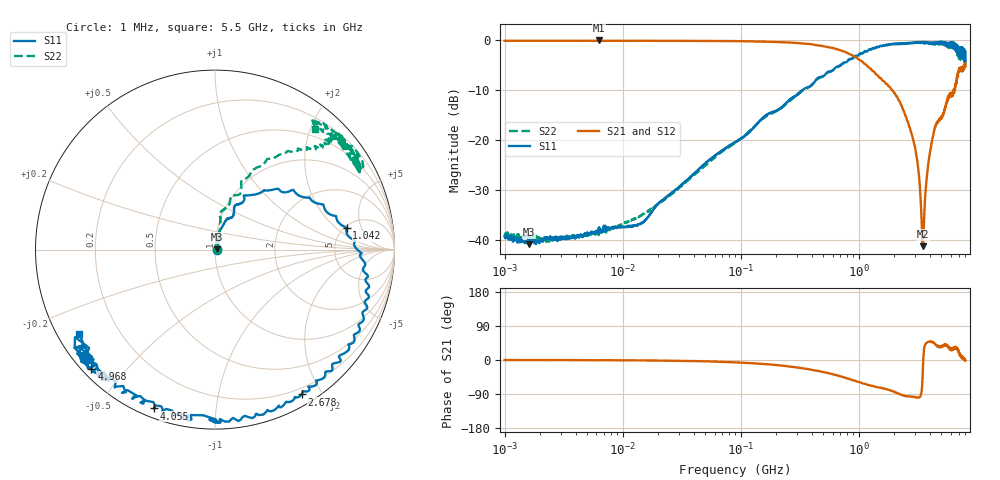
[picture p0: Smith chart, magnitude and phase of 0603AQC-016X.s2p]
!s-Parameter Generated by FASTRON Sdn. Bhd.
!FASTRON P/N : 0603AQC-016X
!Keysight Technologies: E5071C_MY46733604_B.14.02
!Date: Thu Jun 25 13:52:09 2026
!Version  :Rev00  Thu Jun 25 13:52:09 2026
!Data & Calibration Information:
!Freq  S11:SOLT2(ON)  S21:SOLT2(ON)  S12:SOLT2(ON)  S22:SOLT2(ON)
!PortZ  Port1:50+j0  Port2:50+j0
!When reading reference impedance value at option line is always used.
! Remarks : This data is being provided solely for informational purposes.
# Hz S dB R 50
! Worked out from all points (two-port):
!   1601 points, 1 MHz to 8 GHz, reference 50 ohm
!   highest |S21| = -0.03 dB at 6.268 MHz (marker M1); lowest = -41.2 dB at 3.487 GHz (marker M2)
!   |S21| within 3 dB of the highest: start of sweep to 884.1 MHz
!   lowest |S11| = -40.8 dB at 1.605 MHz (marker M3), VSWR 1.02, Z = 50.9 + j0.0931 ohm
!   |S11| at or under -10 dB: start of sweep to 332.3 MHz
!   |S22| runs from -40.5 to -0.3 dB; largest |S21 - S12| = 0.019
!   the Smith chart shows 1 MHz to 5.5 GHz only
!   S11 on the Smith chart (normalised r, x): 1 MHz: 1.02, +0.00; 1.042 GHz: 5.26, +2.79; 2.678 GHz: 0.13, -1.76; 4.055 GHz: 0.04, -0.69; 4.968 GHz: 0.03, -0.40; 5.5 GHz: 0.06, -0.29
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1000000  -39.30 2.3  -0.10 -0.1  -0.09 -0.1  -38.80 4.2
1604653  -40.80 5.8  -0.09 -0.2  -0.09 -0.1  -39.70 0.3
4479405  -39.00 24.4  -0.10 -0.3  -0.10 -0.4  -39.10 26.1
6268472  -37.60 22.1  -0.03 -0.5  -0.16 -1.1  -39.00 27.6
1.406113e7  -36.70 47.4  -0.10 -1.1  -0.11 -1.1  -35.10 49.9
2.00676e7  -32.70 54.0  -0.11 -1.5  -0.11 -1.4  -32.80 64.4
8.994653e7  -20.40 77.1  -0.16 -6.2  -0.17 -6.2  -20.50 75.0
4.006501e8  -9.00 58.5  -0.79 -26.1  -0.80 -26.1  -8.84 66.1
6.624464e8  -5.22 37.1  -1.81 -41.0  -1.81 -41.0  -5.34 60.6
1.041574e9  -2.58 9.2  -4.07 -59.6  -4.08 -59.7  -2.74 50.3
1.7949e9  -0.84 -24.3  -9.23 -78.5  -9.26 -78.8  -0.84 43.8
2.677636e9  -0.54 -59.1  -17.30 -95.8  -17.30 -95.8  -0.55 40.3
3.122398e9  -0.51 -75.8  -24.00 -99.5  -24.00 -99.5  -0.50 42.3
3.385893e9  -0.35 -86.6  -34.50 -87.8  -34.50 -87.7  -0.48 37.7
3.487237e9  -0.39 -89.9  -41.20 -24.3  -41.20 -25.0  -0.47 34.6
4.054764e9  -0.46 -111.0  -21.90 47.7  -21.90 47.5  -0.60 38.1
4.968456e9  -0.38 -136.0  -15.70 36.5  -15.60 36.2  -0.53 34.6
5.500301e9  -1.01 -148.0  -12.50 39.0  -12.50 38.6  -1.16 50.3
6.419251e9  -0.47 -169.0  -10.50 28.8  -10.50 28.4  -1.19 51.8
6.843354e9  -1.65 -168.0  -7.35 31.6  -7.33 31.0  -2.12 69.5
7.383122e9  -2.28 150.0  -5.80 6.0  -5.82 5.2  -3.10 44.0
8e9  -2.24 143.0  -5.18 -1.2  -5.21 -1.9  -3.60 54.9
